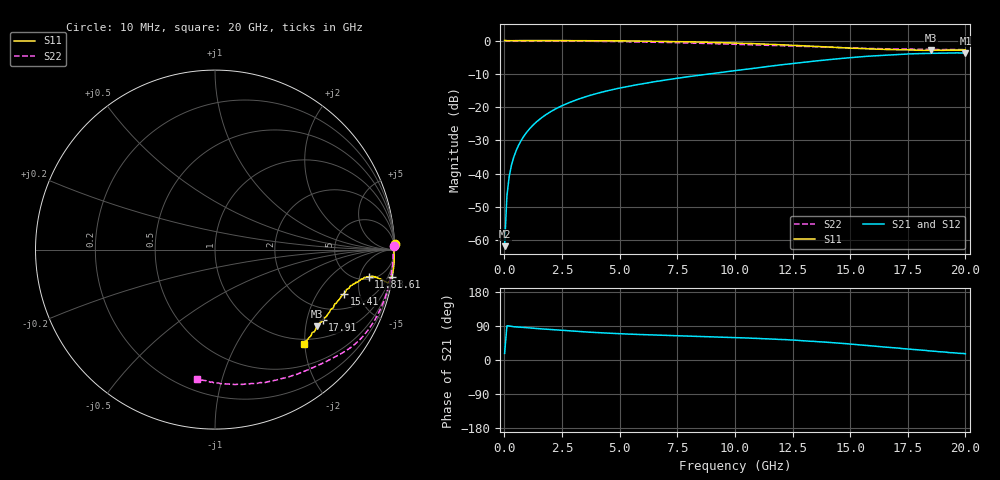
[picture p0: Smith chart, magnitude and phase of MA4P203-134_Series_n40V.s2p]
! AWR Design Environment (9226) Thu Aug 19 14:29:25 2021
! Document = 'n40V'
! nPorts: 2, nXvals: 201
# GHz S DB R 50
!Freq DBS11 AngS11 DBS21 AngS21 DBS12 AngS12 DBS22 AngS22
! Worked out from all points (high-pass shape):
!   201 points, 10 MHz to 20 GHz, reference 50 ohm
!   highest |S21| = -3.71 dB at 20 GHz (marker M1); lowest = -61.9 dB at 10 MHz (marker M2)
!   |S21| within 3 dB of the highest: 12.77 GHz to end of sweep
!   lowest |S11| = -3.0 dB at 18.51 GHz (marker M3), VSWR 5.92, Z = 66.8 - j116 ohm
!   |S11| at or under -10 dB: nowhere
!   |S22| runs from -2.8 to 0.0 dB; largest |S21 - S12| = 0.022
!   S11 on the Smith chart (normalised r, x): 10 MHz: -6, +61; 3.61 GHz: 0, -13; 11.81 GHz: 5.62, -6.94; 15.41 GHz: 3.04, -3.51; 17.91 GHz: 1.54, -2.50; 20 GHz: 0.89, -1.99
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0.01  0.03 1.9  -61.86 17.4  -66.12 -23.2  -0.02 1.3
0.11  -0.04 -0.1  -46.71 90.3  -46.52 89.3  -0.06 -0.7
0.21  -0.04 -0.6  -40.85 89.8  -40.95 88.8  -0.06 -1.4
0.31  -0.02 -0.8  -37.41 88.6  -37.48 88.5  -0.06 -2.0
0.41  -0.02 -1.2  -35.02 87.8  -35.04 87.9  -0.06 -2.7
0.61  -0.01 -1.8  -31.58 86.9  -31.59 87.1  -0.06 -4.0
0.81  -0.01 -2.4  -29.14 86.0  -29.14 86.1  -0.06 -5.3
1.01  -0.01 -2.9  -27.22 85.0  -27.24 85.2  -0.07 -6.5
1.61  0.00 -4.6  -23.25 82.1  -23.25 82.4  -0.08 -10.3
2.41  -0.00 -6.6  -19.91 78.5  -19.91 78.8  -0.13 -15.1
3.41  -0.04 -8.6  -17.15 74.4  -17.15 75.0  -0.19 -20.4
3.61  -0.04 -8.8  -16.72 73.8  -16.72 74.3  -0.20 -21.4
4.91  -0.10 -10.3  -14.43 69.7  -14.43 70.4  -0.31 -27.2
6.71  -0.22 -10.8  -12.18 65.5  -12.16 66.6  -0.52 -33.8
10.01  -0.73 -9.9  -9.04 59.0  -8.99 60.7  -1.12 -45.2
11.81  -1.22 -10.0  -7.47 54.7  -7.39 56.3  -1.51 -53.8
13.41  -1.72 -12.2  -6.22 49.2  -6.11 50.6  -1.87 -63.6
15.41  -2.40 -18.8  -4.91 39.8  -4.84 41.3  -2.30 -77.6
16.71  -2.68 -25.8  -4.36 33.1  -4.31 34.6  -2.49 -85.8
17.91  -2.88 -33.3  -3.94 27.0  -3.97 28.2  -2.64 -91.8
18.51  -2.96 -37.0  -3.86 23.8  -3.89 25.0  -2.71 -93.9
20  -2.79 -46.7  -3.71 16.4  -3.82 18.3  -2.74 -97.7
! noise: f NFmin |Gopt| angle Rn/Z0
0.01  0  1  0  2e-20
2.21  0  1  0  2e-20
4.41  0  1  0  2e-20
6.61  0  1  0  2e-20
8.81  0  1  0  2e-20
11.11  0  1  0  2e-20
13.31  0  1  0  2e-20
15.51  0  1  0  2e-20
17.71  0  1  0  2e-20
20  0  1  0  2e-20
